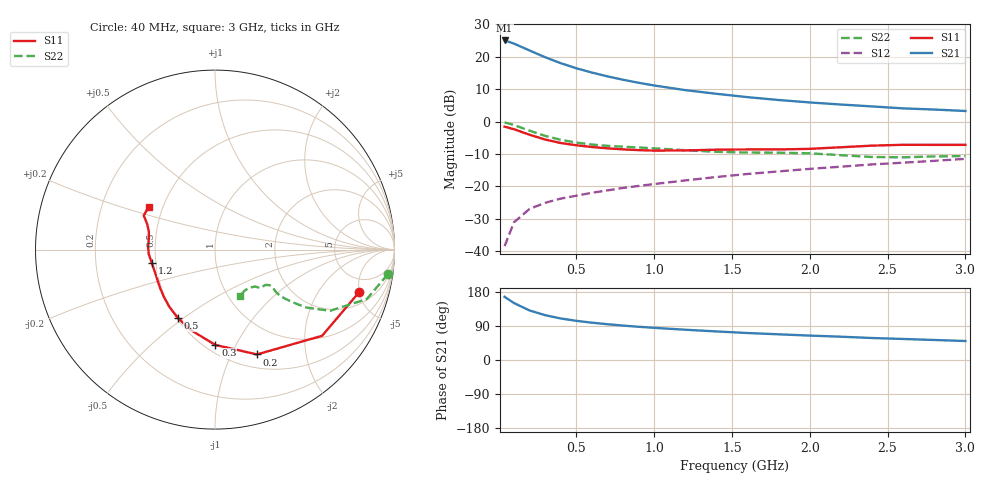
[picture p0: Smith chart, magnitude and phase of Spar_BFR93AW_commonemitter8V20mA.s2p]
! Filename:  BFR93AWG.S2P  Version:  4.0
! NXP part #: BFR93AW  Date: Jun 1994
! Bias condition: Vce=8V, Ic=20mA
#  MHz  S  MA  R  50
! Freq  S11  S21  S12  S22  !GUM [dB]
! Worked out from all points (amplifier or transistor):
!   21 points, 40 MHz to 3 GHz, reference 50 ohm
!   highest |S21| = 25.1 dB at 40 MHz (marker M1)
!   |S21| within 3 dB of that: start of sweep to 196 MHz
!   unconditionally stable (mu >= 1): 983.6 MHz to end of sweep
!   at 300 MHz: K = 0.54, MSG = 22.5 dB, |S12| = -25.0 dB
!   at 1 GHz: K = 1.01, MAG = 14.7 dB, |S12| = -19.3 dB
!   at 3 GHz: K = 1.03, MAG = 6.3 dB, |S12| = -11.5 dB
!   S11 on the Smith chart (normalised r, x): 40 MHz: 3.14, -4.98; 200 MHz: 0.65, -1.26; 300 MHz: 0.56, -0.83; 500 MHz: 0.51, -0.47; 1.2 GHz: 0.47, -0.08; 3 GHz: 0.42, +0.25
40  0.837 -16.5  17.93 166.7  0.012 81.5  0.973 -8.1
100  0.766 -38.8  16.04 150.3  0.028 71.0  0.889 -18.1
200  0.629 -68.2  12.57 130.8  0.045 60.5  0.726 -28.0
300  0.531 -89.8  9.882 118.3  0.056 56.2  0.605 -32.3
400  0.469 -106.3  8.005 109.6  0.065 55.6  0.526 -34.1
500  0.433 -118.6  6.681 103.4  0.072 56.1  0.476 -35.0
600  0.407 -128.9  5.73 98.5  0.08 57.4  0.444 -35.3
700  0.388 -137.2  5.007 94.4  0.087 58.8  0.424 -35.1
800  0.374 -144.6  4.444 90.9  0.095 60.2  0.411 -34.7
900  0.364 -151.3  3.989 87.7  0.102 61.3  0.4 -34.1
1000  0.358 -157.5  3.621 84.9  0.109 62.5  0.388 -33.5
1200  0.36 -168.2  3.071 79.9  0.124 64.3  0.363 -33.1
1400  0.37 -176.2  2.694 75.4  0.14 65.9  0.343 -35.0
1600  0.373 178.2  2.393 71.2  0.156 66.6  0.334 -38.5
1800  0.373 172.1  2.161 67.8  0.171 67.7  0.332 -40.1
2000  0.381 165.1  1.982 64.4  0.187 68.5  0.325 -40.8
2200  0.403 159.5  1.84 61.5  0.202 69.2  0.304 -42.6
2400  0.427 156.0  1.721 58.0  0.219 69.6  0.285 -48.0
2600  0.44 154.5  1.604 55.5  0.233 69.5  0.282 -54.9
2800  0.439 151.4  1.54 52.8  0.249 70.1  0.291 -59.4
3000  0.439 147.2  1.463 50.1  0.267 70.1  0.295 -61.9
